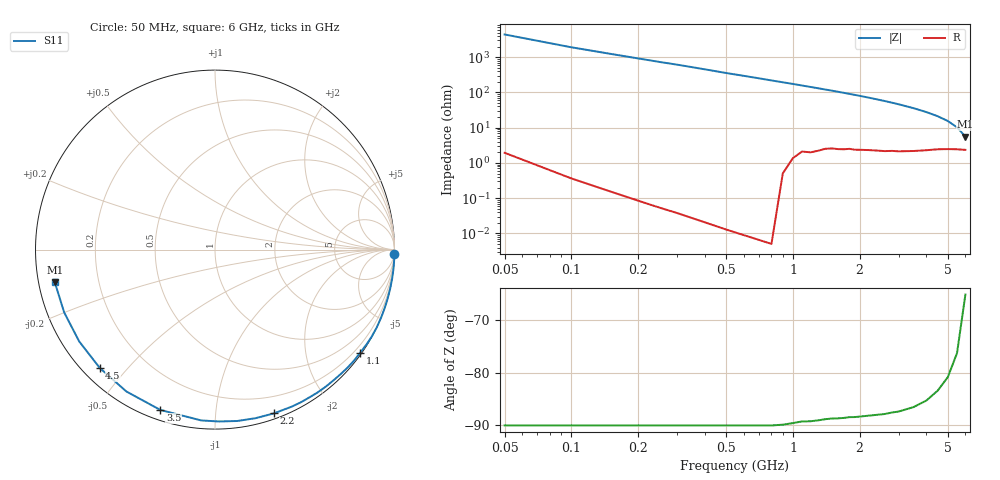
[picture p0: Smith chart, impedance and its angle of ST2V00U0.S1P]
! SIEMENS Discrete & RF Semiconductors
! BA892
! Si PIN Diode in SCD-80
! VR = 2 V
! S-Parameters:  September  1997
# GHz  S  MA  R  50
!  f  S11
! GHz  MAG  ANG
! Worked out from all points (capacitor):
!   34 points, 50 MHz to 6 GHz, reference 50 ohm
!   read as one part to ground: C = 834 fF near 50 MHz
!   lowest |Z| = 5.59 ohm at 6 GHz (marker M1)
!   S11 on the Smith chart (normalised r, x): 50 MHz: 0, -88; 1.1 GHz: 0.04, -3.14; 2.2 GHz: 0.05, -1.42; 3.5 GHz: 0.04, -0.72; 4.5 GHz: 0.05, -0.42; 6 GHz: 0.05, -0.10
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0.05  1 -1.3
0.25  1 -7.8
0.4  1 -12.6
0.5  1 -16.0
0.6  1 -19.2
0.7  1 -22.4
0.8  1 -25.7
0.9  0.9987 -28.9
1  0.9958 -32.0
1.1  0.9923 -35.3
1.2  0.9913 -38.5
1.3  0.9888 -41.7
1.4  0.9854 -44.9
1.6  0.9817 -51.2
1.7  0.9798 -54.4
1.9  0.976 -60.7
2  0.9738 -63.9
2.2  0.9698 -70.2
2.4  0.9661 -76.5
2.6  0.9629 -82.6
2.8  0.9579 -88.7
3  0.9549 -94.6
3.5  0.9439 -108.8
4  0.9321 -122.0
4.5  0.9202 -134.3
5  0.9134 -146.0
5.5  0.9102 -157.4
6  0.9109 -168.4
